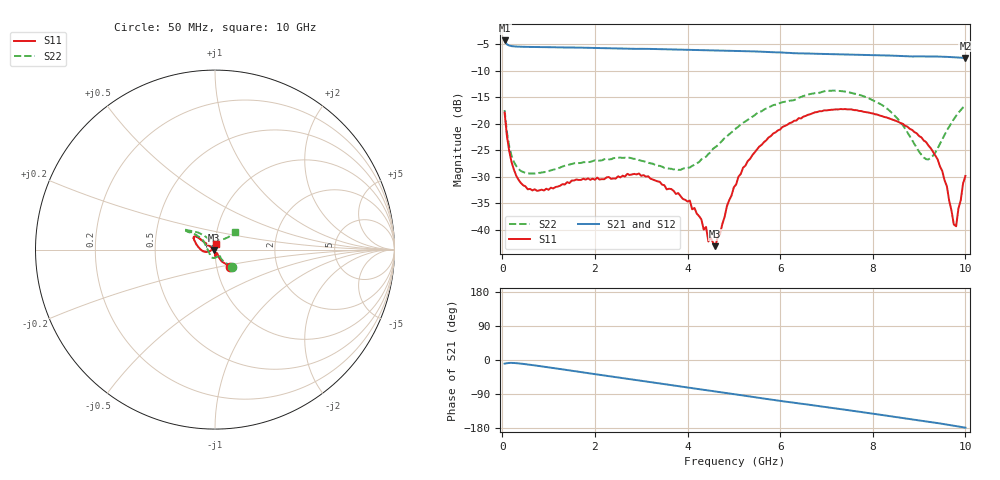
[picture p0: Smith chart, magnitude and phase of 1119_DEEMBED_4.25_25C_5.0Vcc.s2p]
!Hittite Microwave Corp.
!Digital Attenuator/PhaseShifter Rev 1.4.0
!Filename: C:\DATA\DATA\1119_DEEMBED_4.25_25C_5.0Vcc.s2p
!VNA ID: Agilent Technologies,N5224A,MY51441122,A.10.45.03
!Device type:
!2 Port Calibration.
!Temp(C): 25
!Lot Number:
!Serial Number:
!Operator:
!Misc:
!Attenuator:  4.250
# GHZ S DB R 50.0
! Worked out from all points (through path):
!   200 points, 50 MHz to 10 GHz, reference 50 ohm
!   highest |S21| = -4.26 dB at 50 MHz (marker M1); lowest = -7.6 dB at 10 GHz (marker M2)
!   group delay of S21, straight-line fit = 48.4 ps
!   lowest |S11| = -43.1 dB at 4.6 GHz (marker M3), VSWR 1.01, Z = 49.4 - j0.346 ohm
!   |S11| at or under -10 dB: start of sweep to end of sweep
!   |S22| runs from -29.4 to -13.7 dB; largest |S21 - S12| = 0.0018
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0.05  -17.89 -48.2  -4.26 -9.6  -4.26 -9.6  -17.40 -45.0
0.1  -22.29 -60.1  -5.00 -8.5  -5.00 -8.5  -21.59 -54.7
0.2  -27.24 -63.2  -5.33 -7.6  -5.33 -7.6  -26.03 -54.8
0.55  -32.37 -59.4  -5.48 -11.8  -5.47 -11.8  -29.37 -50.5
1.75  -30.37 -88.2  -5.62 -32.7  -5.63 -32.8  -27.26 -80.1
2.95  -29.39 -89.1  -5.84 -53.8  -5.85 -53.8  -26.86 -120.0
3.4  -30.95 -89.8  -5.89 -61.8  -5.90 -61.9  -27.95 -137.0
4.05  -34.49 -85.5  -6.03 -73.4  -6.04 -73.5  -28.24 -174.6
4.4  -39.47 -102.7  -6.11 -79.6  -6.12 -79.7  -26.21 162.4
4.45  -42.22 -113.2  -6.13 -80.5  -6.15 -80.5  -25.70 159.9
4.6  -43.11 -149.9  -6.15 -83.0  -6.17 -83.1  -24.42 151.9
5.05  -31.45 149.5  -6.23 -90.9  -6.25 -91.0  -20.85 141.8
5.2  -28.28 146.7  -6.26 -93.6  -6.28 -93.7  -19.80 141.0
5.75  -22.58 145.4  -6.44 -103.5  -6.45 -103.5  -16.88 142.7
6.7  -18.01 145.1  -6.74 -119.3  -6.76 -119.3  -14.29 146.9
7.5  -17.27 151.1  -6.92 -132.9  -6.93 -132.9  -14.08 145.9
8.35  -18.97 161.4  -7.11 -147.9  -7.11 -147.9  -17.43 134.8
9.2  -24.09 -170.5  -7.28 -162.6  -7.29 -162.6  -26.73 92.6
9.5  -28.90 -164.1  -7.32 -168.4  -7.34 -168.4  -22.94 52.7
9.75  -39.01 147.1  -7.43 -173.5  -7.44 -173.5  -19.13 42.2
9.799999  -39.35 125.7  -7.46 -174.5  -7.47 -174.5  -18.49 41.7
10  -29.85 75.6  -7.57 -178.5  -7.58 -178.5  -16.51 40.5
